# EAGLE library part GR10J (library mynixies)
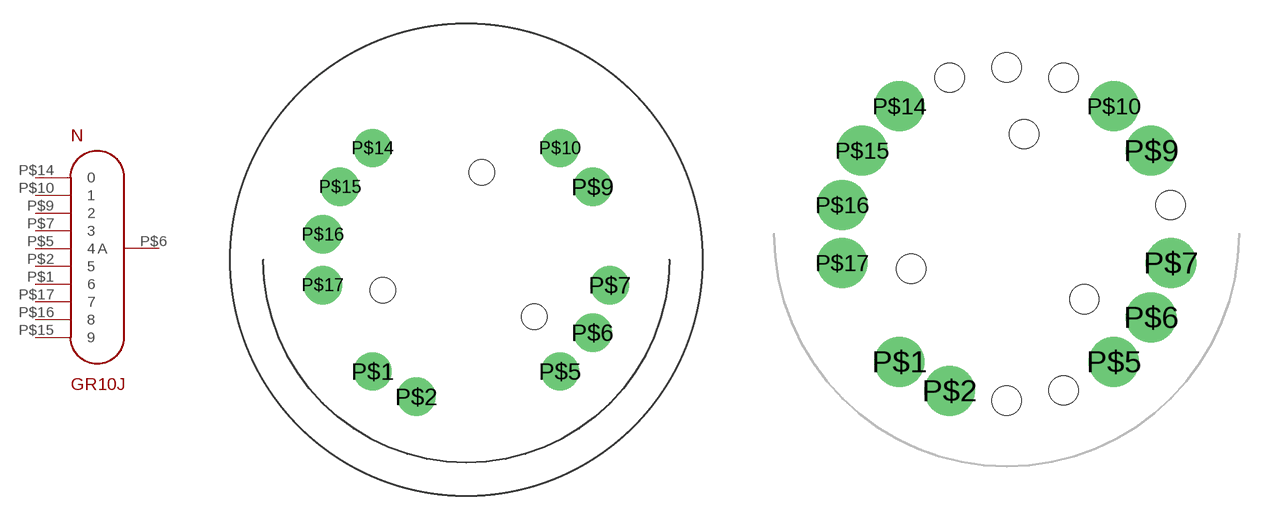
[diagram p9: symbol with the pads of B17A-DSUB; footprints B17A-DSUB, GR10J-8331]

Designator prefix N

## GR10JB17A  [B17A-DSUB]
P$1  6  pas
P$2  5  pas
P$5  4  pas
P$6  A  pas
P$7  3  pas
P$9  2  pas
P$10  1  pas
P$14  0  pas
P$15  9  pas
P$16  8  pas
P$17  7  pas

## GR10J  [GR10J-8331]
Pads as for B17A-DSUB

## Footprint B17A-DSUB (pad centres in mm)
drill 1.6: P$1 -5.861,-6.985; P$2 -3.119,-8.569; P$5 5.861,-6.985; P$6 7.897,-4.559; P$7 8.98,-1.583; P$9 7.897,4.559; P$10 5.861,6.985; P$14 -5.861,6.985; P$15 -7.897,4.559; P$16 -8.98,1.583; P$17 -8.98,-1.583
hole 1.6 at 0.964,5.466
hole 1.6 at -5.215,-1.898
hole 1.6 at 4.251,-3.567

## Footprint GR10J-8331 (pad centres in mm)
drill 1.829: P$1 -5.861,-6.985; P$2 -3.119,-8.569; P$5 5.861,-6.985; P$6 7.897,-4.559; P$7 8.98,-1.583; P$9 7.897,4.559; P$10 5.861,6.985; P$14 -5.861,6.985; P$15 -7.897,4.559; P$16 -8.98,1.583; P$17 -8.98,-1.583
hole 1.6 at 0.964,5.466
hole 1.6 at -5.215,-1.898
hole 1.6 at 4.251,-3.567
hole 1.6 at 8.962,1.58
hole 1.6 at 3.112,8.551
hole 1.6 at 0,9.1
hole 1.6 at -3.112,8.551
hole 1.6 at 0,-9.1
hole 1.6 at 3.112,-8.551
